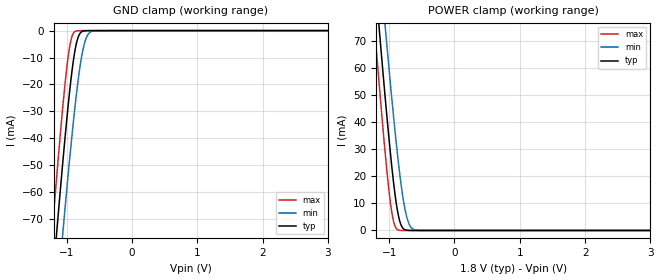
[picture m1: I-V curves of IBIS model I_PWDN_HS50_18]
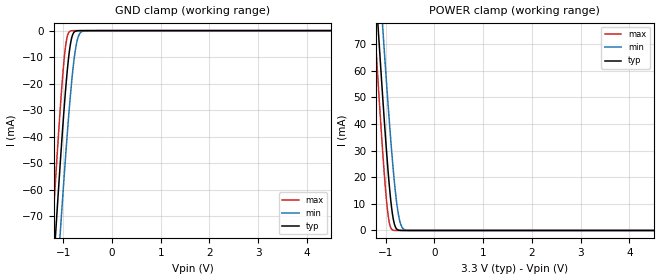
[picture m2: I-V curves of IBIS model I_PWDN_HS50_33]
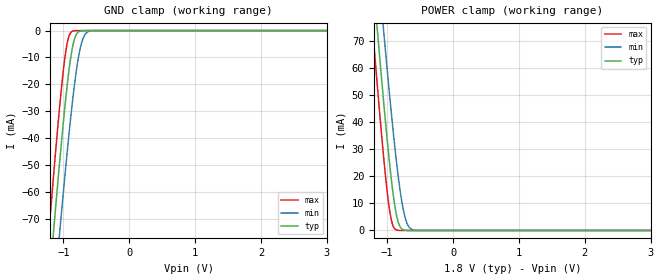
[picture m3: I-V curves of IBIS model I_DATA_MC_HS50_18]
| Texas Instruments Incorporated
| DS90UB914Q
| 10-100MHz 10/12 Bit DC Balanced FPD Link III Serializer and Deserializer
| with Bi-Directional Control Channel
| Marketing part#   Voltage Range   Package-type   Temperature
| DS90UB914AQ1SQE   1.71V - 3.6V   48-Pin LLP   -40 to 105C
| DS90UB914AQ1SQ   1.71V - 3.6V   48-Pin LLP   -40 to 105C
| DS90UB914AQ1SQX   1.71V - 3.6V   48-Pin LLP   -40 to 105C
[IBIS Ver]   4.0
[File name]   ds90ub914a-q1.ibs
[File Rev]   1.0
[Date]   04/11/2012
[Source]   Model built from TISPICE simulations at:
   Texas Instruments Incorporated.
   WEBENCH DESIGN CENTER
   12500 TI Blvd
   Dallas, TX -75243
   For Support e-mail: elab_scm_ibis@list.ti.com
[Notes]   Rev 1.0: 04/11/2012
   - Initial version of the IBIS model
   - All models are generated in Spectre
   - ccomp is listed in numerical order, for PVT information,
   please check notes above ccomp keyword for each model
   - All non-monotonic warnings can be ignored as per buffer behavior
[Disclaimer] This product is designed as an aid for customers of Texas Instruments.
   No warranties, either expressed or implied, with respect to this third
   party software (if any) or with respect to its fitness for any
   particular purpose is claimed by Texas Instruments or the author. The
   software (if any) is provided solely on an "as is" basis. The entire
   risk as to its quality and performance is with the customer
[Copyright]   (C)Copyright 2012 Texas Instruments Incorporated.
   All rights reserved.
|   DS90UB914A-Q1
[Component]  DS90UB914A-Q1
[Manufacturer]  Texas Instruments, Inc.
[Package]   | 6.0x6.0x0.5mm 48-pin LLP package
|   typ   min   max
R_pkg   0   0   0
L_pkg   0   0   0
C_pkg   0   0   0
[Pin]   signal_name   model_name   R_pin   L_pin   C_pin
1   SDA   IO_SMBUS_HS50
2   SCL   IO_SMBUS_HS50
3   VDDSSCG   POWER
4   OSS_SEL   IO_DATA_50_HS50
5   OEN   IO_DATA_50_HS50
6   BISTEN   I_PWDN_HS50
7   VDDIO3   POWER
8   PCLK   IO_CLK_100M_HS50
9   VSYNC   IO_DATA_50_ATP_HS50
10   HSYNC   IO_DATA_50_ATP_HS50
11   ROUT[11]   IO_DATA_50_HS50
12   ROUT[10]   IO_DATA_50_HS50
13   ROUT[9]   IO_DATA_50_HS50
14   ROUT[8]   IO_DATA_50_HS50
15   ROUT[7]   IO_DATA_50_HS50
16   ROUT[6]   IO_DATA_50_HS50
17   VDDD   POWER
18   ROUT[5]   IO_DATA_50_HS50
19   ROUT[4]   IO_DATA_50_HS50
20   VDDIO2   POWER
21   ROUT[3]   IO_DATA_50_HS50
22   ROUT[2]   IO_DATA_50_HS50
23   ROUT[1]   IO_DATA_50_HS50
24   ROUT[0]   IO_DATA_50_HS50
25   GPIO[3]   IO_DATA_50_ATP_HS50
26   GPIO[2]   IO_DATA_50_ATP_HS50
27   GPIO[1]   IO_DATA_50_ATP_HS50
28   GPIO[0]   IO_DATA_50_ATP_HS50
29   VDDIO1   POWER
30   PDB   I_PWDN_HS50
31   VDDCML1   POWER
32   RIN+   NC
33   RIN-   NC
34   IDX[1]   NC
35   IDX[0]   NC
36   VDDR   POWER
37   MODE   NC
38   CMLOUTP   NC
39   CMLOUTN   NC
40   VDDCML0   POWER
41   RIN0+   NC
42   RIN0-   NC
43   RES   NC
44   RES   NC
45   VDDPLL   POWER
46   SEL   I_DATA_MC_HS50
47   PASS   IO_DATA_50_HS50
48   LOCK   IO_DATA_50_ATP_HS50
49   DAP   GND
[Package Model] LLP48 DS90UB914
[Model Selector]   I_PWDN_HS50
I_PWDN_HS50_33   I_PWDN_HS50 input with VDD=3.3V
I_PWDN_HS50_18   I_PWDN_HS50 input with VDD=1.8V
[Model Selector]   I_DATA_MC_HS50
I_DATA_MC_HS50_33   I_DATA_MC_HS50 input with VDD=3.3V
I_DATA_MC_HS50_18   I_DATA_MC_HS50 input with VDD=1.8V
[Model Selector]   IO_DATA_50_ATP_HS50
IO_DATA_50_ATP_HS50_33   IO_DATA_50_ATP_HS50 with VDD=3.3V
IO_DATA_50_ATP_HS50_18   IO_DATA_50_ATP_HS50 with VDD=1.8V
[Model Selector]   IO_DATA_50_HS50
IO_DATA_50_HS50_33   IO_DATA_50_HS50 with VDD=3.3V
IO_DATA_50_HS50_18   IO_DATA_50_HS50 with VDD=1.8V
[Model Selector]   IO_SMBUS_HS50
IO_SMBUS_HS50_33   IO_SMBUS_HS50 with VDD=3.3V
IO_SMBUS_HS50_18   IO_SMBUS_HS50 with VDD=1.8V
[Model Selector]   IO_CLK_100M_HS50
IO_CLK_100M_HS50_33   IO_CLK_100M_HS50 with VDD=3.3V
IO_CLK_100M_HS50_18   IO_CLK_100M_HS50 with VDD=1.8V
[Define Package Model]  LLP48 DS90UB914
[Manufacturer]  Unknown
[OEM]  Unknown
[Description]  None
[Number Of Pins]  49
[Pin Numbers]
|Pin Num   Terminal Name
1   | L1:W1
2   | L2:W2
3   | L3:3
4   | L4:W5
5   | L5:W6
6   | L6:W7
7   | L7:7
8   | L8:W10
9   | L9:W11
10   | L10:W12
11   | L11:W13
12   | L12:W14
13   | L13:W15
14   | L14:W16
15   | L15:W17
16   | L16:W18
17   | L17:17
18   | L18:W22
19   | L19:W23
20   | L20:20
21   | L21:W27
22   | L22:W28
23   | L23:W29
24   | L24:W30
25   | L25:W31
26   | L26:W32
27   | L27:W33
28   | L28:W34
29   | L29:29
30   | L30:W37
31   | L31:31
32   | L32:W40
33   | L33:W41
34   | L34:W42
35   | L35:W43
36   | L36:36
37   | L37:W47
38   | L38:W48
39   | L39:W49
40   | L40:40
41   | L41:W52
42   | L42:W53
43   | L43:W54
44   | L44:W55
45   | L45:45
46   | L46:W58
47   | L47:W59
48   | L48:W60
49   | LDAP:49
[Model Data]
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[End Model Data]
[End Package Model]
| Models and submodels in the file (12): I_PWDN_HS50_18 (Input), I_PWDN_HS50_33 (Input), I_DATA_MC_HS50_18 (Input), I_DATA_MC_HS50_33 (Input), IO_DATA_50_ATP_HS50_33 (I/O), IO_DATA_50_ATP_HS50_18 (I/O), IO_DATA_50_HS50_33 (I/O), IO_DATA_50_HS50_18 (I/O), IO_SMBUS_HS50_33 (I/O_open_drain), IO_SMBUS_HS50_18 (I/O_open_drain), IO_CLK_100M_HS50_33 (I/O), IO_CLK_100M_HS50_18 (I/O)
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|   Model I_PWDN_HS50_18
[Model]   I_PWDN_HS50_18
Model_type   Input
Vinl = 0.63V
Vinh = 1.17V
|   typ   min   max
|   (nom)   (weak)   (fast)
C_comp   0.5928pF   0.5928pF   0.5928pF
[Voltage Range]   1.800V   1.710V   1.890V
[Temperature Range]   25.0   105.0   -40.0
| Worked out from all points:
|   GND clamp passes 1 mA (typ) near -0.79 V on its own axis
|   POWER clamp passes 1 mA (typ) near -0.79 V on its own axis
[GND Clamp]
|   Voltage   I(typ)   I(min)   I(max)
-1.8V     -270.9mA   -291mA     -255.6mA
-1.228V   -97.1mA    -122.7mA   -76.77mA
-1.201V   -89.21mA   -115mA     -68.71mA
-1.147V   -73.63mA   -99.73mA   -52.87mA
-1.055V   -48.06mA   -74.39mA   -27.51mA
-957.6mV  -23.54mA   -48.82mA   -6.663mA
-871.2mV  -7.328mA   -28.21mA   -335.2uA
-811.8mV  -1.781mA   -16.28mA   -25.67uA
-741.6mV  -161.6uA   -6.205mA   -6.921uA
-682.2mV  -20.1uA    -1.83mA    -5.854uA
-601.2mV  -4.02uA    -199.2uA   -5.127uA
3.595V    6.712uA    3.483uA    12.03uA
[POWER Clamp]
|   Voltage   I(typ)   I(min)   I(max)
-1.8V     270.2mA    290.2mA    254.8mA
-1.228V   96.77mA    122.3mA    76.49mA
-1.201V   88.9mA     114.6mA    68.45mA
-1.147V   73.36mA    99.39mA    52.65mA
-1.055V   47.86mA    74.11mA    27.37mA
-957.6mV  23.41mA    48.61mA    6.6mA
-871.2mV  7.262mA    28.06mA    325.8uA
-811.8mV  1.758mA    16.17mA    20.65uA
-741.6mV  156.5uA    6.146mA    2.661uA
-682.2mV  17.07uA    1.807mA    2.011uA
-601.2mV  1.608uA    195uA      1.824uA
3.595V    0A         0A         0A
|   Model I_PWDN_HS50_33
[Model]   I_PWDN_HS50_33
Model_type   Input
Vinl = 0.8V
Vinh = 2.0V
|   typ   min   max
|   (nom)   (weak)   (fast)
C_comp   0.5928pF   0.5928pF   0.5928pF
[Voltage Range]   3.300V   3.000V   3.600V
[Temperature Range]   25.0   105.0   -40.0
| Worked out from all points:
|   GND clamp passes 1 mA (typ) near -0.79 V on its own axis
|   POWER clamp passes 1 mA (typ) near -0.79 V on its own axis
[GND Clamp]
|   Voltage   I(typ)   I(min)   I(max)
-3.3V     -740.6mA   -745.8mA   -738.2mA
-1.231V   -98.06mA   -123.6mA   -77.76mA
-1.221V   -95.16mA   -120.8mA   -74.79mA
-1.171V   -80.77mA   -106.7mA   -60.12mA
-1.142V   -72.26mA   -98.38mA   -51.49mA
-1.063V   -50.17mA   -76.5mA    -29.54mA
-953.7mV  -22.65mA   -47.84mA   -6.095mA
-914.1mV  -14.38mA   -38.09mA   -1.938mA
-854.7mV  -5.279mA   -24.66mA   -158.3uA
-735.9mV  -131.2uA   -5.62mA    -6.724uA
-597.3mV  -3.893uA   -177.7uA   -5.09uA
6.59V     7.865uA    3.955uA    14.61uA
[POWER Clamp]
|   Voltage   I(typ)   I(min)   I(max)
-3.3V     739mA      744.2mA    736.5mA
-1.231V   97.8mA     123.3mA    77.52mA
-1.221V   94.9mA     120.5mA    74.56mA
-1.171V   80.54mA    106.4mA    59.92mA
-1.142V   72.04mA    98.11mA    51.31mA
-1.063V   50mA       76.28mA    29.42mA
-953.7mV  22.55mA    47.67mA    6.048mA
-914.1mV  14.3mA     37.95mA    1.916mA
-854.7mV  5.24mA     24.55mA    149.8uA
-735.9mV  126.1uA    5.58mA     498.8nA
-597.3mV  637nA      174.2uA    50.05nA
6.59V     0A         0A         0A
|   Model I_DATA_MC_HS50_18
[Model]   I_DATA_MC_HS50_18
Model_type   Input
Vinl = 0.63V
Vinh = 1.17V
|   typ   min   max
|   (nom)   (weak)   (fast)
C_comp   0.5928pF   0.5928pF   0.5928pF
[Voltage Range]   1.800V   1.710V   1.890V
[Temperature Range]   25.0   105.0   -40.0
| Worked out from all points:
|   GND clamp passes 1 mA (typ) near -0.79 V on its own axis
|   POWER clamp passes 1 mA (typ) near -0.79 V on its own axis
[GND Clamp]
|   Voltage   I(typ)   I(min)   I(max)
-1.8V     -271mA     -291mA     -255.6mA
-1.228V   -97.13mA   -122.7mA   -76.8mA
-1.201V   -89.24mA   -115mA     -68.74mA
-1.147V   -73.66mA   -99.76mA   -52.9mA
-1.055V   -48.09mA   -74.42mA   -27.54mA
-957.6mV  -23.57mA   -48.85mA   -6.691mA
-871.2mV  -7.355mA   -28.24mA   -349uA
-811.8mV  -1.796mA   -16.31mA   -35.11uA
-741.6mV  -166.7uA   -6.23mA    -13.16uA
-682.2mV  -22.73uA   -1.842mA   -9.797uA
-601.2mV  -4.882uA   -201.7uA   -6.456uA
3.595V    0A         0A         0A
[POWER Clamp]
|   Voltage   I(typ)   I(min)   I(max)
-1.8V     270.2mA    290.2mA    254.9mA
-1.228V   96.77mA    122.3mA    76.49mA
-1.201V   88.91mA    114.6mA    68.45mA
-1.147V   73.37mA    99.4mA     52.66mA
-1.055V   47.86mA    74.12mA    27.37mA
-957.6mV  23.41mA    48.61mA    6.602mA
-871.2mV  7.263mA    28.06mA    324uA
-811.8mV  1.758mA    16.17mA    18.49uA
-741.6mV  155.5uA    6.146mA    576.2nA
-682.2mV  16.1uA     1.807mA    26.76nA
-601.2mV  704.2nA    194.6uA    0A
3.595V    0A         0A         0A
